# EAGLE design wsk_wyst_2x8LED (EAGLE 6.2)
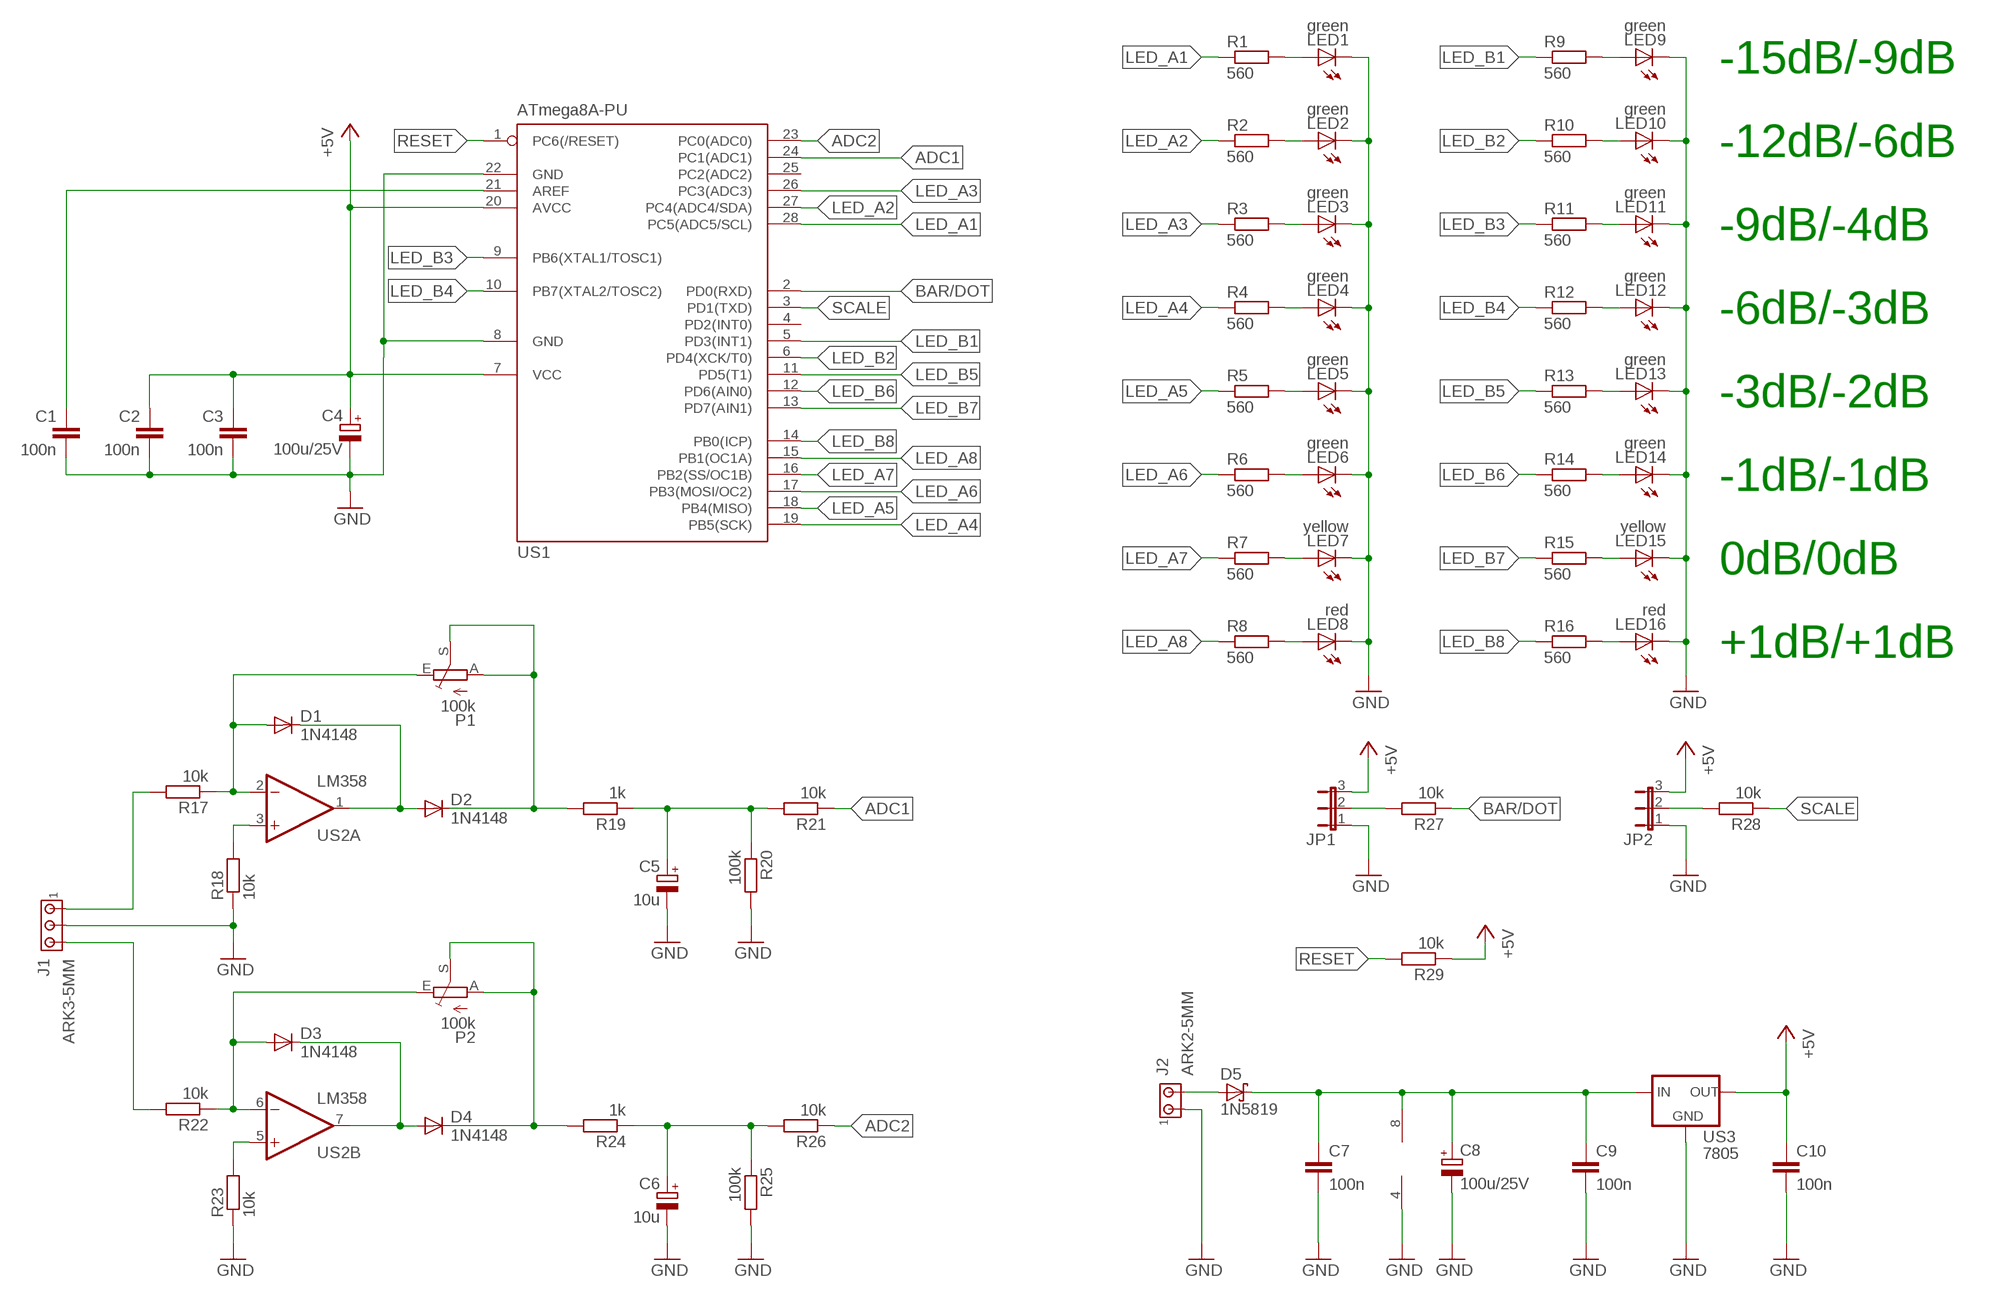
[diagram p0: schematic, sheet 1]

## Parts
C1  100n  C-EU050-025X075  [C050-025X075]
C2  100n  C-EU050-025X075  [C050-025X075]
C3  100n  C-EU050-025X075  [C050-025X075]
C4  100u/25V  CPOL-EUTT2D5L  [TT2D5L]
C5  10u  CPOL-EUTT2D5L  [TT2D5L]
C6  10u  CPOL-EUTT2D5L  [TT2D5L]
C7  100n  C-EU050-025X075  [C050-025X075]
C8  100u/25V  CPOL-EUTT2D5L  [TT2D5L]
C9  100n  C-EU050-025X075  [C050-025X075]
C10  100n  C-EU050-025X075  [C050-025X075]
D1  1N4148  1N4148DO35-7  [DO35-7]
D2  1N4148  1N4148DO35-7  [DO35-7]
D3  1N4148  1N4148DO35-7  [DO35-7]
D4  1N4148  1N4148DO35-7  [DO35-7]
D5  1N5819  1N5819-T  [DO41-7.6]
J1  ARK3-5MM  [3PIN-5MM]
J2  ARK2-5MM  [2PIN-5MM]
JP1  JP2E  [JP2]
JP2  JP2E  [JP2]
LED1  green  LED5MM  [LED5MM]
LED2  green  LED5MM  [LED5MM]
LED3  green  LED5MM  [LED5MM]
LED4  green  LED5MM  [LED5MM]
LED5  green  LED5MM  [LED5MM]
LED6  green  LED5MM  [LED5MM]
LED7  yellow  LED5MM  [LED5MM]
LED8  red  LED5MM  [LED5MM]
LED9  green  LED5MM  [LED5MM]
LED10  green  LED5MM  [LED5MM]
LED11  green  LED5MM  [LED5MM]
LED12  green  LED5MM  [LED5MM]
LED13  green  LED5MM  [LED5MM]
LED14  green  LED5MM  [LED5MM]
LED15  yellow  LED5MM  [LED5MM]
LED16  red  LED5MM  [LED5MM]
P1  100k  TRIM_EU-CA6V  [CA6V]
P2  100k  TRIM_EU-CA6V  [CA6V]
R1  560  R-EU_0207/7  [0207/7]
R2  560  R-EU_0207/7  [0207/7]
R3  560  R-EU_0207/7  [0207/7]
R4  560  R-EU_0207/7  [0207/7]
R5  560  R-EU_0207/7  [0207/7]
R6  560  R-EU_0207/7  [0207/7]
R7  560  R-EU_0207/7  [0207/7]
R8  560  R-EU_0207/7  [0207/7]
R9  560  R-EU_0207/7  [0207/7]
R10  560  R-EU_0207/7  [0207/7]
R11  560  R-EU_0207/7  [0207/7]
R12  560  R-EU_0207/7  [0207/7]
R13  560  R-EU_0207/7  [0207/7]
R14  560  R-EU_0207/7  [0207/7]
R15  560  R-EU_0207/7  [0207/7]
R16  560  R-EU_0207/7  [0207/7]
R17  10k  R-EU_0207/7  [0207/7]
R18  10k  R-EU_0207/7  [0207/7]
R19  1k  R-EU_0207/7  [0207/7]
R20  100k  R-EU_0207/7  [0207/7]
R21  10k  R-EU_0207/7  [0207/7]
R22  10k  R-EU_0207/7  [0207/7]
R23  10k  R-EU_0207/7  [0207/7]
R24  1k  R-EU_0207/7  [0207/7]
R25  100k  R-EU_0207/7  [0207/7]
R26  10k  R-EU_0207/7  [0207/7]
R27  10k  R-EU_0207/7  [0207/7]
R28  10k  R-EU_0207/7  [0207/7]
R29  10k  R-EU_0207/7  [0207/7]
US1  ATmega8A-PU  MEGA8-P  [DIL28-3]
US2  LM358  LM358N  [DIL08]
US3  7805  78XXS  [78XXS]

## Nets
+5V: C2.1 C3.1 C4.+ C10.1 JP1.3 JP2.3 R29.1 US1.7(VCC) US1.20(AVCC) US3.OUT
ADC1: R21.1 US1.24(PC1(ADC1))
ADC2: R26.1 US1.23(PC0(ADC0))
BAR/DOT: R27.1 US1.2(PD0(RXD))
GND: C1.2 C2.2 C3.2 C4.- C5.- C6.- C7.2 C8.- C9.2 C10.2 J1.P$2 J2.P$1 JP1.1 JP2.1 LED1.K(C) LED2.K(C) LED3.K(C) LED4.K(C) LED5.K(C) LED6.K(C) LED7.K(C) LED8.K(C) LED9.K(C) LED10.K(C) LED11.K(C) LED12.K(C) LED13.K(C) LED14.K(C) LED15.K(C) LED16.K(C) R18.1 R20.2 R23.1 R25.2 US1.8(GND) US1.22(GND) US2.4(P:V-) US3.GND
LED_A1: R1.1 US1.28(PC5(ADC5/SCL))
LED_A2: R2.1 US1.27(PC4(ADC4/SDA))
LED_A3: R3.1 US1.26(PC3(ADC3))
LED_A4: R4.1 US1.19(PB5(SCK))
LED_A5: R5.1 US1.18(PB4(MISO))
LED_A6: R6.1 US1.17(PB3(MOSI/OC2))
LED_A7: R7.1 US1.16(PB2(SS/OC1B))
LED_A8: R8.1 US1.15(PB1(OC1A))
LED_B1: R9.1 US1.5(PD3(INT1))
LED_B2: R10.1 US1.6(PD4(XCK/T0))
LED_B3: R11.1 US1.9(PB6(XTAL1/TOSC1))
LED_B4: R12.1 US1.10(PB7(XTAL2/TOSC2))
LED_B5: R13.1 US1.11(PD5(T1))
LED_B6: R14.1 US1.12(PD6(AIN0))
LED_B7: R15.1 US1.13(PD7(AIN1))
LED_B8: R16.1 US1.14(PB0(ICP))
N$1: LED1.A R1.2
N$2: LED2.A R2.2
N$3: LED3.A R3.2
N$4: LED4.A R4.2
N$5: LED5.A R5.2
N$6: LED6.A R6.2
N$7: LED7.A R7.2
N$8: LED8.A R8.2
N$9: R18.2 US2.3(A:+IN)
N$17: LED9.A R9.2
N$18: LED10.A R10.2
N$19: LED11.A R11.2
N$20: LED12.A R12.2
N$21: LED13.A R13.2
N$22: LED14.A R14.2
N$23: LED15.A R15.2
N$24: LED16.A R16.2
N$40: C1.1 US1.21(AREF)
N$41: JP1.2 R27.2
N$42: D1.A P1.E R17.1 US2.2(A:-IN)
N$43: D1.C D2.A US2.1(A:OUT)
N$44: D2.C P1.A P1.S R19.2
N$45: R23.2 US2.5(B:+IN)
N$46: D3.A P2.E R22.1 US2.6(B:-IN)
N$47: D3.C D4.A US2.7(B:OUT)
N$48: D4.C P2.A P2.S R24.2
N$49: J1.P$3 R22.2
N$50: J1.P$1 R17.2
N$51: C6.+ R24.1 R25.1 R26.2
N$52: C5.+ R19.1 R20.1 R21.2
N$53: JP2.2 R28.2
N$54: D5.A J2.P$2
N$55: C7.1 C8.+ C9.1 D5.C US2.8(P:V+) US3.IN
RESET: R29.2 US1.1(PC6(/RESET))
SCALE: R28.1 US1.3(PD1(TXD))
Unconnected: US1.4(PD2(INT0)) US1.25(PC2(ADC2))

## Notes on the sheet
- -15dB/-9dB
- -12dB/-6dB
- -9dB/-4dB
- -6dB/-3dB
- -3dB/-2dB
- -1dB/-1dB
- 0dB/0dB
- +1dB/+1dB

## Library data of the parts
C1-C3 C7 C9 C10 = rcl:C-EU: CAPACITOR, European symbol
C4-C6 C8 = rcl:CPOL-EU: POLARIZED CAPACITOR, European symbol
D1-D4 = diode:1N4148: DIODE
D5 = diode:1N581*: 1.0A SCHOTTKY BARRIER RECTIFIER
J1 = zlacza_futrzak:ARK3: ARK 3 Raster 5mm i 3,5mm
J2 = zlacza_futrzak:ARK2: ARK 2
JP1 JP2 = jumper:JP2E: JUMPER
LED1-LED16 = led:LED: LED
P1 P2 = pot:TRIM_EU-: POTENTIOMETER
R1-R29 = rcl:R-EU_: RESISTOR, European symbol
US1 = atmel:MEGA8-P: MICROCONTROLLER 8 Kbytes FLASH, 1 kbytes SRAM, 512 bytes EEPROM, USART, 4-channel 10 bit ADC, 2-channel 8 bit ADC Pin compatible with Atmega48, ATMega88, ATMega168 Source: avr.lbr; OC_FARNELL: unknown; OC_NEWARK: unknown
US2 = linear:LM358: OP AMP also LM158; LM258; LM2904 Source: http://cache.national.com/ds/LM/LM158.pdf
US3 = v-reg:78XXS: VOLTAGE REGULATOR

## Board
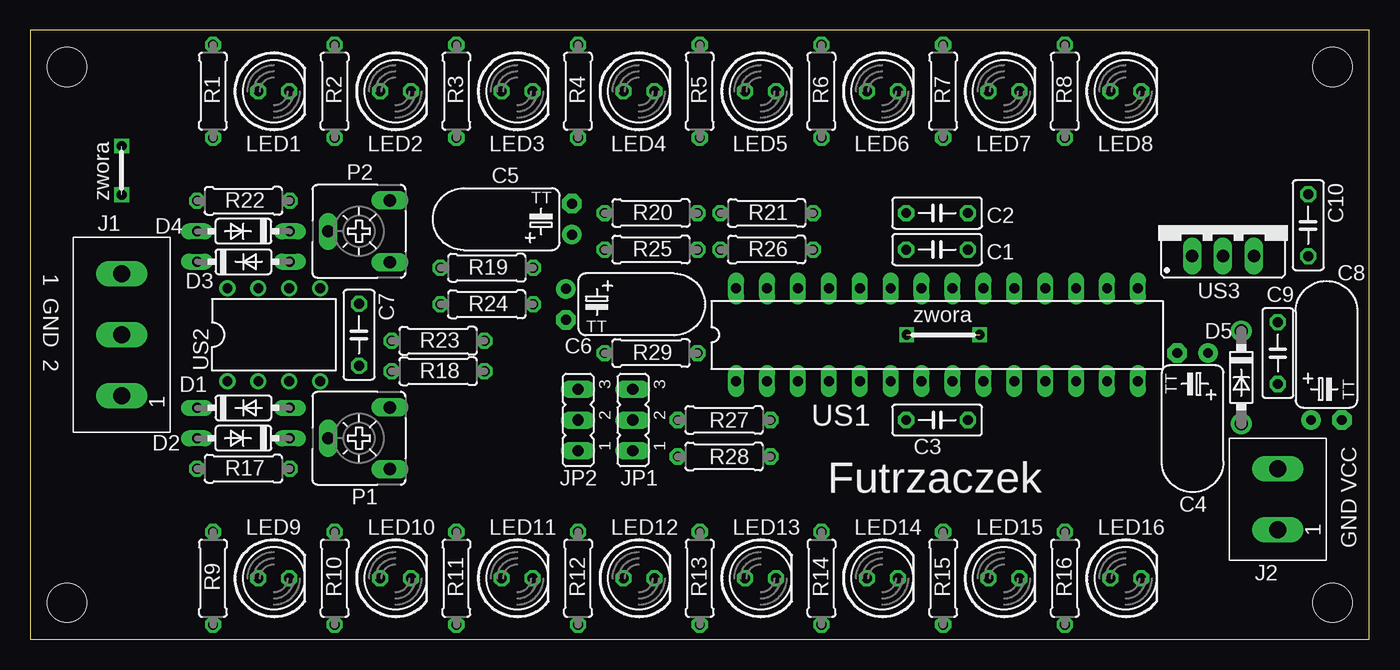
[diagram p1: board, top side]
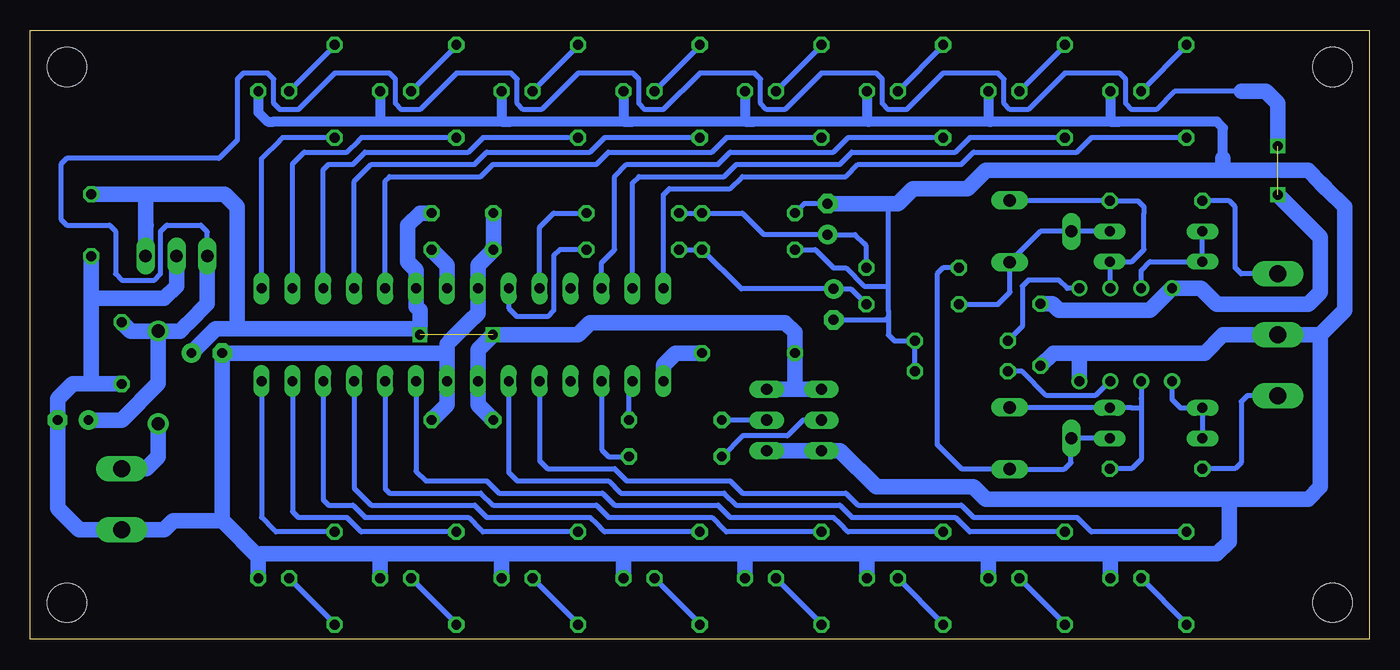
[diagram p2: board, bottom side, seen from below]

Size 110 x 50 mm. Coordinates in mm from the lower left corner, seen from the top.
Outline: 0,0 110,0 110,50 0,50 0,0
Copper layers (1*16): Top 0.035mm / dielectric 1.5mm / Bottom 0.035mm
Design rules: minimum track width 10mil, minimum drill 24mil, track to track 8mil, track to pad 8mil, pad to pad 8mil, via to via 8mil, smd to smd 8mil, copper to edge 20mil, drill to drill 8mil, minimum pad ring 10mil, minimum via ring 8mil, stop-mask expansion 4mil, vias tented up to drill 0mil, thermal gap 10mil
Holes 3.2 mm at 3,3 3,47 107,3 107,47

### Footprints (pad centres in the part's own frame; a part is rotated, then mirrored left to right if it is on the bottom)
C050-025X075 = drill 0.813 octagon: 1 -2.54,0; 2 2.54,0
TT2D5L = drill 0.813 pad 1.6: + -1.27,0 | drill 0.813 pad 1.6 octagon: - 1.27,0
DO35-7 = drill 0.813 long: A 3.81,0; C -3.81,0
DO41-7.6 = drill 1.1 pad 1.7: A 3.81,0; C -3.81,0
3PIN-5MM = drill 1.4 long: P$1 -5,0; P$2 0,0; P$3 5,0
2PIN-5MM = drill 1.4 long: P$1 -2.5,0; P$2 2.5,0
JP2 = drill 0.914 long: 1 -2.54,0; 2 0,0; 3 2.54,0
LED5MM = drill 0.813 octagon: A -1.27,0; K 1.27,0
CA6V = drill 1.016 long: A -2.54,-2.54; E 2.54,-2.54; S 0,2.54
0207/7 = drill 0.813 octagon: 1 -3.81,0; 2 3.81,0
DIL28-3 = drill 0.813 long: 1 -16.51,-3.81; 2 -13.97,-3.81; 3 -11.43,-3.81; 4 -8.89,-3.81; 5 -6.35,-3.81; 6 -3.81,-3.81; 7 -1.27,-3.81; 8 1.27,-3.81; 9 3.81,-3.81; 10 6.35,-3.81; 11 8.89,-3.81; 12 11.43,-3.81; 13 13.97,-3.81; 14 16.51,-3.81; 15 16.51,3.81; 16 13.97,3.81; 17 11.43,3.81; 18 8.89,3.81; 19 6.35,3.81; 20 3.81,3.81; 21 1.27,3.81; 22 -1.27,3.81; 23 -3.81,3.81; 24 -6.35,3.81; 25 -8.89,3.81; 26 -11.43,3.81; 27 -13.97,3.81; 28 -16.51,3.81
DIL08 = drill 0.813 pad 1.27: 1 -3.81,-3.81; 2 -1.27,-3.81; 3 1.27,-3.81; 4 3.81,-3.81; 5 3.81,3.81; 6 1.27,3.81; 7 -1.27,3.81; 8 -3.81,3.81
78XXS = drill 1.016 long: GND 0,-2.54; IN -2.54,-2.54; OUT 2.54,-2.54

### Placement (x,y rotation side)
C1  74.5,32 180 top
C2  74.5,35 180 top
C3  74.5,18 0 top
C4  95.5,23.5 180 top
C5  44.5,34.5 90 top
C6  44,27.5 270 top
C7  27,25 270 top
C8  106.5,18 0 top
C9  102.5,23.5 270 top
C10  105,34 270 top
D1  17.5,19 0 top
D2  17.5,16.5 180 top
D3  17.5,31 0 top
D4  17.5,33.5 180 top
D5  99.5,21.5 270 top
J1  7.5,25 90 top
J2  102.5,11.5 90 top
JP1  49.5,18 90 top
JP2  45,18 90 top
LED1  20,45 0 top
LED2  30,45 0 top
LED3  40,45 0 top
LED4  50,45 0 top
LED5  60,45 0 top
LED6  70,45 0 top
LED7  80,45 0 top
LED8  90,45 0 top
LED9  20,5 0 top
LED10  30,5 0 top
LED11  40,5 0 top
LED12  50,5 0 top
LED13  60,5 0 top
LED14  70,5 0 top
LED15  80,5 0 top
LED16  90,5 0 top
P1  27,16.5 90 top
P2  27,33.5 90 top
R1  15,45 90 top
R2  25,45 90 top
R3  35,45 90 top
R4  45,45 90 top
R5  55,45 90 top
R6  65,45 90 top
R7  75,45 90 top
R8  85,45 90 top
R9  15,5 270 top
R10  25,5 270 top
R11  35,5 270 top
R12  45,5 270 top
R13  55,5 270 top
R14  65,5 270 top
R15  75,5 270 top
R16  85,5 270 top
R17  17.5,14 180 top
R18  33.5,22 180 top
R19  37.5,30.5 180 top
R20  51,35 180 top
R21  60.5,35 180 top
R22  17.5,36 180 top
R23  33.5,24.5 180 top
R24  37.5,27.5 180 top
R25  51,32 180 top
R26  60.5,32 180 top
R27  57,18 180 top
R28  57,15 180 top
R29  51,23.5 0 top
US1  74.5,25 0 top
US2  20,25 0 top
US3  98,34 0 top

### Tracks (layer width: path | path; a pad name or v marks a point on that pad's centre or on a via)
+5V  (via drill 0.8)  (1 unrouted)
  Bottom 1.27: C2.1 78,35 79,34 79,31 78.31,30.31 US1.20 78.31,27.31 78,27 78,25.5 | C3.1 73.23,19.27 US1.7 73.23,23.77 v72,25 65,25 64,26 48,26 47.19,25.19 R29.1 47.19,20.85 47.5,20.54 | 93,25.5 78,25.5 | 78,25.5 v78,25 | JP2.3 47.5,20.54 | 47.5,20.54 48.96,20.54 49,20.5 49.46,20.5 JP1.3 | 93,25.5 94.77,25.5 C4.+ | US3.OUT 100.54,33.96 | 100.54,33.96 100.5,34 | 93,25.5 93,35.5 94.04,36.54 100.5,36.54 | C10.1 100.5,36.54 | 100.54,33.96 100.54,36.5 100.5,36.54
ADC1
  Bottom 0.406: US1.24 68.15,33.85 67,35 R21.1
ADC2
  Bottom 0.406: R26.1 66.5,32 67,31.5 67,27 67.5,26.5 70,26.5 70.69,27.19 US1.23
BAR/DOT
  Bottom 0.406: R27.1 60.81,20.91 US1.2
GND
  Bottom 0.406: C6.- 40.27,26.23 39.77,26.23 39.5,26.5 | 39.5,29 39.5,27 39.5,26.5 | C5.- 46.42,35.77 R20.2 | R25.2 45.5,32 44,30.5 43,30.5 41.5,29 39.5,29 | R18.1 R23.1 39,24.5 39.5,25 39.5,26.5 | 39.5,29 39.5,35.77
  Bottom 0.813: 12,39.5 12,42 12.5,42.5 20.5,42.5 | 20.5,42.5 31,42.5 | 31,42.5 41,42.5 | 41,42.5 50.5,42.5 | 50.5,42.5 60.5,42.5 | 60.5,42.5 70.5,42.5 | 70.5,42.5 81.5,42.5 | 81.5,42.5 90,42.5 90.5,42.5 91.27,43.27 LED8.K | LED1.K 21.27,42.5 20.5,42.5 | LED2.K 31.27,42.5 31,42.5 | LED3.K 41.27,42.5 41,42.5 | LED4.K 51.27,42.5 50.5,42.5 | LED5.K 61.27,42.5 60.5,42.5 | LED6.K 71.27,42.5 70.5,42.5 | LED7.K 81.27,42.5 81.5,42.5
  Bottom 1.27: C2.2 C1.2 73.23,30.73 US1.22 73.23,26.77 73.5,26.5 73.73,26.27 75.5,24.5 75.77,24.23 75.77,23.5 | 75.77,23.5 US1.8 75.77,19.27 C3.2 | 75.77,23.5 85.5,23.5 C4.- 94.23,9.73 | LED16.K 91.27,6.77 | 91.27,6.77 94,9.5 94.23,9.73 | LED9.K 21.27,6.27 21.27,6.73 21,7 | 31,7 22,7 21,7 | 31,7 41.5,7 | 41.5,7 51.5,7 | 51.5,7 61,7 | 61,7 71.5,7 | 71.5,7 81.5,7 | 81.5,7 91.04,7 91.27,6.77 | LED15.K 81.27,6.77 81.5,7 | LED14.K 71.27,6.77 71.5,7 | LED13.K 61.27,6.73 61,7 | LED12.K 51.27,6.77 51.5,7 | LED11.K 41.27,6.77 41.5,7 | LED10.K 31.27,6.73 31,7 | JP1.1 JP2.1 43.46,15.46 40.5,12.5 32.5,12.5 31.5,11.5 23,11.5 11.5,11.5 | 94.23,9.73 98.27,9.73 99,9 J2.P$1 106,9 107,10 107.77,10.77 C8.- 107.77,19.73 107.5,20 106.54,20.96 105,20.96 | C9.2 105,20.96 | 105,20.96 105,27.5 105,28 | 105,28 C10.2 | 105,28 102,28 99,28 98,29 US3.GND | C5.- 39.5,35.77 38.73,35.77 37.5,37 33,37 31.5,38.5 12,38.5 | 12,38.5 5,38.5 4,37.5 3.5,37 2,35.5 2,27 4,25 | 12,39.5 12,38.5 | 23.5,23.5 24.5,23.5 25.96,23.5 C7.2 | 23.5,23.5 13.5,23.5 12,25 J1.P$2 5,25 4,25 | US2.4 23.81,23.19 23.5,23.5 | 11.5,11.5 5,11.5 4,12.5 4,23 4,25 | 21,7 12.5,7 11.5,8 11.5,11.5
LED_A1
  Bottom 0.406: US1.28 57.99,36.51 57.5,37 52.5,37 51.5,38 43,38 42,39 33.5,39 32.5,40 24,40 | 24,40 23.5,40.5 | R1.1 22.81,41.19 24,40
LED_A2
  Bottom 0.406: US1.27 60.53,37.47 60,38 53,38 52,39 43.5,39 42.5,40 34,40 33.5,40.5 32.81,41.19 R2.1
LED_A3
  Bottom 0.406: R3.1 42.81,41.19 44,40 52.5,40 53.5,39 61,39 62,38 62,32 63.07,30.93 US1.26
LED_A4
  Bottom 0.406: US1.19 80.85,37.65 80.5,38 73,38 72,39 63.5,39 62.5,40 54,40 53,41 52.81,41.19 R4.1
LED_A5
  Bottom 0.406: US1.18 83.39,37.61 82,39 73.5,39 72.5,40 64,40 62.81,41.19 R5.1
LED_A6
  Bottom 0.406: US1.17 85.93,38.57 85.5,39 83.5,39 82.5,40 74,40 73,41 72.81,41.19 R6.1
LED_A7
  Bottom 0.406: US1.16 88.47,39.03 88,39.5 87.5,40 84,40 83,41 82.81,41.19 R7.1
LED_A8
  Bottom 0.406: US1.15 91.01,39.49 89.5,41 89.31,41.19 R8.1
LED_B1
  Bottom 0.406: US1.5 68.15,14.65 67.5,14 62,14 61,13 52.5,13 51.5,12 43,12 42,11 33.5,11 32.5,10 24,10 23.5,9.5 22.81,8.81 R9.1
LED_B2
  Bottom 0.406: US1.6 70.69,13.69 70,13 62.5,13 61.5,12 53,12 52,11 43.5,11 42.5,10 34,10 33.5,9.5 32.81,8.81 R10.1
LED_B3
  Bottom 0.406: US1.9 78.31,13.81 77.5,13 72.5,13 71.5,12 63,12 62,11 53.5,11 52.5,10 44,10 43.5,9.5 42.81,8.81 R11.1
LED_B4
  Bottom 0.406: US1.10 80.85,12.35 80.5,12 73,12 72,11 63.5,11 62.5,10 54,10 53,9 52.81,8.81 R12.1
LED_B5
  Bottom 0.406: US1.11 83.39,12.39 82,11 73.5,11 72.5,10 64,10 63.5,9.5 62.81,8.81 R13.1
LED_B6
  Bottom 0.406: US1.12 85.93,11.43 85.5,11 83.5,11 82.5,10 74,10 73,9 72.81,8.81 R14.1
LED_B7
  Bottom 0.406: US1.13 88.47,10.47 88,10 84,10 83,9 82.81,8.81 R15.1
LED_B8
  Bottom 0.406: US1.14 91.01,10.01 90,9 89.81,8.81 R16.1
N$1
  Bottom 0.406: R1.2 15,48.73 LED1.A
N$2
  Bottom 0.406: R2.2 25,48.73 LED2.A
N$3
  Bottom 0.406: R3.2 35,48.73 LED3.A
N$4
  Bottom 0.406: R4.2 45,48.73 LED4.A
N$5
  Bottom 0.406: R5.2 55,48.73 LED5.A
N$6
  Bottom 0.406: R6.2 65,48.73 LED6.A
N$7
  Bottom 0.406: R7.2 75,48.73 LED7.A
N$8
  Bottom 0.406: R8.2 85,48.73 LED8.A
N$9
  Bottom 0.406: US2.3 21.31,21.19 22.5,20 26.5,20 28.5,22 R18.2
N$17
  Bottom 0.406: R9.2 15,1.27 LED9.A
N$18
  Bottom 0.406: R10.2 25,1.27 LED10.A
N$19
  Bottom 0.406: R11.2 35,1.27 LED11.A
N$20
  Bottom 0.406: R12.2 45,1.27 LED12.A
N$21
  Bottom 0.406: R13.2 55,1.27 LED13.A
N$22
  Bottom 0.406: R14.2 65,1.27 LED14.A
N$23
  Bottom 0.406: R15.2 75,1.27 LED15.A
N$24
  Bottom 0.406: R16.2 85,1.27 LED16.A
N$40
  Bottom 1.27: US1.21 75.77,30.73 C1.1
N$41
  Bottom 0.406: JP1.2 R27.2
N$42
  Bottom 0.406: P1.E 21.35,19.04 D1.A 19.5,19 18.73,19 | US2.2 18.73,19.77 18.73,19 | 18.73,19 18.73,14.77 19.5,14 R17.1
N$43
  Bottom 0.406: US2.1 16.19,19.69 15.5,19 D1.C D2.A
N$44
  Bottom 0.406: R19.2 35,30.5 35.5,30 35.5,16 33.5,14 29.58,14 P1.A 25.04,13.96 24.5,14.5 24.5,16.46 P1.S D2.C
N$45
  Bottom 0.406: US2.5 24.81,28.81 25.5,29.5 28,29.5 28.5,29 28.5,25.69 R23.2
N$46
  Bottom 0.406: US2.6 21.27,30.96 D3.A 19.5,31 18.5,32 18.5,35 18.5,35.5 19,36 R22.1 21.35,36.04 P2.E
N$47
  Bottom 0.406: US2.7 18.73,30.27 18,31 D3.C D4.A
N$48
  Bottom 0.406: R24.2 30.5,27.5 29.5,28.5 29.5,30.92 P2.A 27,33.5 P2.S D4.C
N$49
  Bottom 0.406: J1.P$3 10.5,30 11,30.5 11,35.5 11.5,36 R22.2
N$50
  Bottom 0.406: J1.P$1 10,20 10.5,19.5 10.5,14.5 11,14 R17.2
N$51
  Bottom 0.406: R26.2 R25.1 51.58,28.77 C6.+ 42.58,28.77 R24.1
N$52
  Bottom 0.406: R21.2 R20.1 51.5,35 50,33.5 49.73,33.23 C5.+ 42.23,33.23 41.5,32.5 41.31,32.31 R19.1
N$53
  Bottom 0.406: R28.2 51.49,16.7 47.8,16.7 47.5,17 46.5,18 JP2.2
N$54
  Bottom 1.27: D5.A 99.5,15 100.5,14 J2.P$2
N$55  (via drill 0.8)  (1 unrouted)
  Bottom 0.406: 10.5,45 16,45 17.5,43.5 19.5,43.5 20,44 20,46 20.5,46.5 25,46.5 28,43.5 29.5,43.5 30,44 30,46 30.5,46.5 35,46.5 38,43.5 39.5,43.5 40,44 40,46 40.5,46.5 45,46.5 48,43.5 49.5,43.5 50,44 50,46 50.5,46.5 55,46.5 58,43.5 59.5,43.5 60,44 60,46 60.5,46.5 65,46.5 68,43.5 69.5,43.5 70,44 70,46 70.5,46.5 75,46.5 78,43.5 79.5,43.5 80,44 80,46 80.5,46.5 85,46.5 88,43.5 89.5,43.5 90,44 90,46 90.5,46.5 92.5,46.5 93,46 93,42 93,41 94,40 94.5,39.5 107,39.5 107.5,39 107.5,34.5 107,34 103.5,34 103,33.5 103,30 102.5,29.5 99.8,29.5 99.3,30 99.3,33.5 98.8,34 96,34 95.46,33.46 US3.IN
  Bottom 1.27: C7.1 26.04,27.54 25.5,27 18,27 US2.8 13.81,28.81 12.5,27.5 5,27.5 4,28.5 4,33 5.5,34.5 v7.5,36.5 | C8.+ 103,18 102.5,18 99.5,21 99.5,21.5 D5.C | D5.C 97.69,25.31 97.19,25.81 97,26 95.46,27.54 US3.IN | D5.C 101.77,25.31 C9.1 | v7.5,40.5 7.5,44 8.5,45 10.5,45
RESET
  Bottom 1.27: R29.2 57,23.5 57.5,23 57.99,22.51 US1.1
SCALE
  Bottom 0.406: US1.3 63.07,15.57 62.5,15 R28.1

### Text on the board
tPlace: zwora | 1 GND 2 | zwora | Futrzaczek | GND VCC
